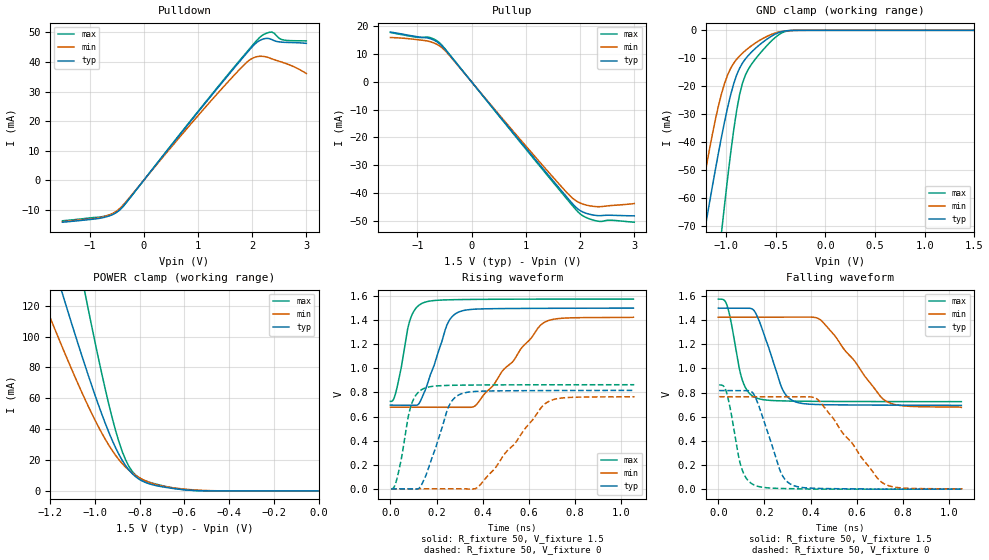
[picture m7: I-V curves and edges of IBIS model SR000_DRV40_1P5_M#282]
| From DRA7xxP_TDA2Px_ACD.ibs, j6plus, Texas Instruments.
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| Model based on original model for DDR_DIFFIOPB_V
|   Sub model SR000_DRV40_1P5
[model]   SR000_DRV40_1P5_M#282
|[Description]  [1.5V-I/O-X-X]
|   , ,
|[Input Load]
|[Output Drive]
|Voltage   1.5V
|Mode   I/O
Model_type   I/O
Polarity   Non-Inverting
Enable   Active-Low
Vinl =  0.65
Vinh =  0.85
Cref =  15.0000pF
Rref =  100.0000M
Vref =  0V
Vmeas =  0.75
C_comp   2p   2p   2p
[Model Spec]
Vinl   0.65   0.6125   0.6875
Vinh   0.85   0.8125   0.8875
[Receiver Thresholds]
Tslew_ac = 0.5n
Vth = 0.75
Vth_max = 0.7875
Vth_min = 0.675
Vinh_ac = 0.175
Vinh_dc = 0.1
Vinl_ac = -0.175
Vinl_dc = -0.1
[Temperature Range]   25   125   -40
[Voltage Range]   1.5   1.425   1.575
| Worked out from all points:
|   slope of the pulldown table from 0 to 0.225 V, typ, clamps not added: 43 ohm
|   slope of the pullup table from 0 to 0.225 V, typ, clamps not added: 41.7 ohm
|   GND clamp passes 1 mA (typ) near -0.48 V on its own axis
|   POWER clamp passes 1 mA (typ) near -0.62 V on its own axis
|   rising waveform, R_fixture 50, V_fixture 1.5: 20-80 % time 82.9ps typ, 189ps min, 50.6ps max; typ from 0.695 V to 1.5 V
|   rising waveform, R_fixture 50, V_fixture 0: 20-80 % time 83ps typ, 185ps min, 50.5ps max; typ from 0 V to 0.817 V
|   falling waveform, R_fixture 50, V_fixture 1.5: 20-80 % time 83.7ps typ, 176ps min, 52.3ps max; typ from 1.5 V to 0.695 V
|   falling waveform, R_fixture 50, V_fixture 0: 20-80 % time 83.6ps typ, 179ps min, 51.7ps max; typ from 0.817 V to 0 V
[POWER_clamp]
-1.5V     302.8mA    223.9mA    484.4mA
-1.242V   174.3mA    127.3mA    279.1mA
-1.136V   123.3mA    89.68mA    196.8mA
-1.045V   81.65mA    59.62mA    128.8mA
-1.03V    75mA       54.92mA    117.8mA
-939.4mV  38.44mA    29.91mA    56.84mA
-893.9mV  23.93mA    20.41mA    32.31mA
-848.5mV  13.61mA    13.43mA    15.91mA
-803mV    7.623mA    8.663mA    8.564mA
-712.1mV  3.022mA    3.561mA    3.877mA
-575.8mV  470.5uA    872uA      449uA
0V        112.6nA    435.6nA    613.8nA
[Pulldown]
-1.5V     -14.18mA   -14.05mA   -13.7mA
-727.3mV  -12.54mA   -12.27mA   -12.15mA
-545.5mV  -11.35mA   -10.95mA   -11.1mA
-409.1mV  -9.378mA   -8.925mA   -9.416mA
1.227V    28.16mA    26.58mA    28.43mA
1.818V    41.23mA    38.42mA    41.56mA
2V        45.11mA    41.2mA     45.49mA
2.182V    47.62mA    41.92mA    48.94mA
2.273V    47.99mA    41.65mA    49.78mA
2.364V    47.57mA    41.06mA    50.1mA
2.545V    46.7mA     39.96mA    47.58mA
3V        46.28mA    36.09mA    47.12mA
[Pullup]
-1.5V     17.97mA    16.01mA    17.82mA
-1V       16.28mA    15.23mA    16.1mA
-772.7mV  15.66mA    14.54mA    16.02mA
-590.9mV  13.75mA    12.97mA    14.08mA
-409.1mV  9.799mA    9.534mA    9.955mA
1.409V    -33.42mA   -32.26mA   -33.94mA
1.773V    -41.87mA   -40.19mA   -42.52mA
1.909V    -44.87mA   -42.6mA    -45.68mA
2.091V    -47.15mA   -44.23mA   -48.65mA
2.318V    -48.13mA   -44.93mA   -50.11mA
2.591V    -48.02mA   -44.49mA   -49.82mA
3V        -48.22mA   -43.8mA    -50.51mA
[GND_clamp]
-1.5V     -133.6mA   -115.7mA   -234.3mA
-1.288V   -87.29mA   -67.59mA   -156.8mA
-1.197V   -68.11mA   -48.64mA   -124.4mA
-1.045V   -38.25mA   -22.77mA   -72.51mA
-1.015V   -32.88mA   -19.1mA    -62.74mA
-954.5mV  -23.3mA    -13.72mA   -44.4mA
-863.6mV  -13.6mA    -9.192mA   -23.11mA
-803mV    -10.18mA   -7.193mA   -15.89mA
-681.8mV  -5.771mA   -4.027mA   -9.287mA
-500mV    -1.264mA   -914.7uA   -2.429mA
-348.5mV  -52.39uA   -75.11uA   -85.87uA
1.5V      112.6nA    528.1nA    514.5nA
[Ramp]
dV/dt_f 0.48364903/83.821371p 0.44912812/0.17636424n 0.50998143/52.340509p
dV/dt_r 0.49180675/83.243552p 0.46129703/0.18594643n 0.51998788/50.619034p
R_load = 50
[Rising Waveform]
R_fixture = 50
V_fixture = 1.5
V_fixture_min = 1.425
V_fixture_max = 1.575
0s        694.7mV    677.7mV    726mV
26.2ps    694mV      677.6mV    819.5mV
86ps      693.6mV    677.6mV    1.407V
119.7ps   699.3mV    677.6mV    1.517V
140.8ps   774mV      677.6mV    1.543V
246.1ps   1.365V     677.4mV    1.569V
297.3ps   1.469V     676.9mV    1.571V
371.2ps   1.492V     696mV      1.572V
671ps     1.498V     1.386V     1.575V
1.053ns   1.5V       1.425V     1.575V
[Rising Waveform]
R_fixture = 50
V_fixture = 0
V_fixture_min = 0
V_fixture_max = 0
3.612ps   0V         0V         0V
30.99ps   0V         0V         103.4mV
89.21ps   0V         0V         688.8mV
122ps     0V         0V         803.5mV
144.9ps   72.96mV    0V         832.7mV
250.3ps   672.5mV    0V         858.6mV
302.1ps   784.8mV    0V         860.5mV
384.4ps   810mV      23.87mV    862mV
683.8ps   815.7mV    723.3mV    863.8mV
1.056ns   817.1mV    766.1mV    864.1mV
[Falling Waveform]
R_fixture = 50
V_fixture = 1.5
V_fixture_min = 1.425
V_fixture_max = 1.575
0s        1.5V       1.425V     1.575V
40.52ps   1.5V       1.425V     1.507V
91.44ps   1.5V       1.425V     996.8mV
107.8ps   1.5V       1.425V     883.5mV
163.8ps   1.451V     1.425V     756.6mV
274.7ps   841.1mV    1.425V     731.6mV
327ps     729mV      1.425V     729.6mV
446.7ps   700.5mV    1.396V     727.3mV
730.7ps   696.3mV    725mV      725.7mV
1.053ns   694.7mV    677.7mV    725.4mV
[Falling Waveform]
R_fixture = 50
V_fixture = 0
V_fixture_min = 0
V_fixture_max = 0
3.612ps   817.1mV    766.1mV    864.1mV
37.75ps   817.3mV    766.2mV    787.9mV
87.13ps   816.8mV    766.2mV    278.2mV
102.3ps   816.8mV    766.2mV    165.9mV
155.8ps   779.5mV    766.2mV    33.95mV
270.3ps   141.5mV    766.2mV    5.695mV
320.4ps   34.44mV    765.9mV    3.63mV
433.6ps   6.028mV    738.2mV    0V
718.1ps   0V         44.47mV    0V
1.056ns   0V         0V         0V
